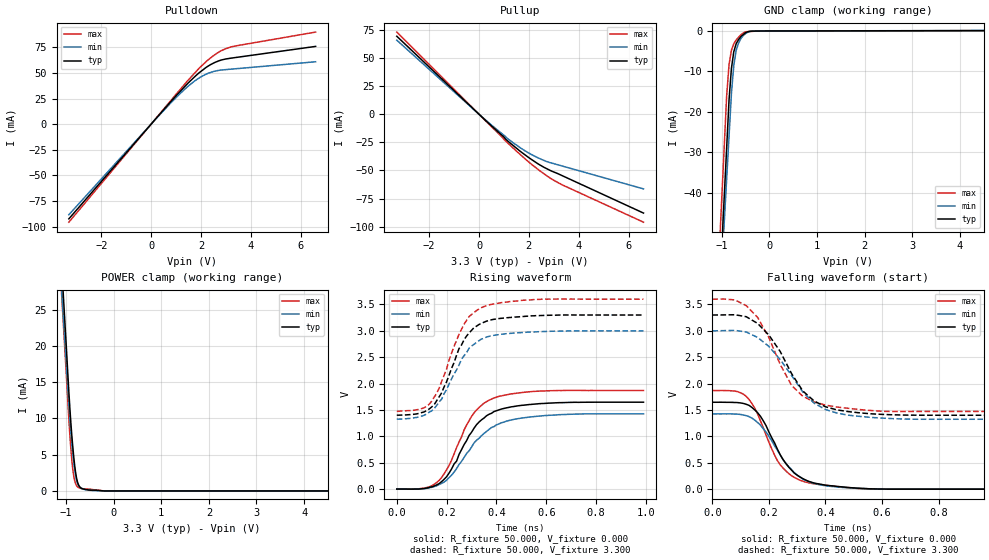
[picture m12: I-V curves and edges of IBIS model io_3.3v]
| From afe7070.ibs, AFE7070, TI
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[Model]   io_3.3v
Model_type I/O
Vinl=1.000E+00
Vinh=2.300E+00
Vref=0.000E+00
Rref=1.000E+06
Cref=0.000E+00
Vmeas=1.650E+00
C_comp   4.3600E-13   4.0000E-13   4.7200E-13
[Voltage Range]   3.300E+00   3.000E+00   3.600E+00
[POWER Clamp Reference]   3.300E+00   3.000E+00   3.600E+00
[GND Clamp Reference]   0.000E+00   0.000E+00   0.000E+00
[Pullup Reference]   3.300E+00   3.000E+00   3.600E+00
[Pulldown Reference]   0.000E+00   0.000E+00   0.000E+00
[Temperature Range]   25   85  -40
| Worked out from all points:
|   slope of the pulldown table from 0 to 0.495 V, typ, clamps not added: 35.8 ohm
|   slope of the pullup table from 0 to 0.495 V, typ, clamps not added: 48.5 ohm
|   GND clamp passes 1 mA (typ) near -0.56 V on its own axis
|   POWER clamp passes 1 mA (typ) near -0.75 V on its own axis
|   rising waveform, R_fixture 50.000, V_fixture 0.000: 20-80 % time 128ps typ, 149ps min, 118ps max; typ from 0 V to 1.65 V
|   falling waveform, R_fixture 50.000, V_fixture 0.000: 20-80 % time 108ps typ, 115ps min, 101ps max; typ from 1.65 V to 0 V
|   rising waveform, R_fixture 50.000, V_fixture 3.300: 20-80 % time 109ps typ, 118ps min, 108ps max; typ from 1.4 V to 3.3 V
|   falling waveform, R_fixture 50.000, V_fixture 3.300: 20-80 % time 137ps typ, 148ps min, 125ps max; typ from 3.3 V to 1.4 V
[GND Clamp]
-3.3V     -598.8mA   -544.4mA   -610mA
-900mV    -29mA      -36.72mA   -16.07mA
-850mV    -17.13mA   -26.15mA   -8.365mA
-800mV    -9.303mA   -15.57mA   -4.792mA
-750mV    -5.128mA   -8.543mA   -3.172mA
-700mV    -3.157mA   -4.777mA   -2.199mA
-650mV    -2.135mA   -2.997mA   -1.566mA
-600mV    -1.36mA    -1.854mA   -932uA
-500mV    -399uA     -615.8uA   -196.2uA
-400mV    -50.66uA   -108.8uA   -123.4uA
-175mV    -5.712uA   -4.952uA   -12.66uA
6.6V      127.9uA    166.2uA    116.8uA
[Power Clamp]
-3.3V     283.4mA    254.2mA    276.7mA
-1.02V    22.77mA    20.23mA    18.9mA
-920mV    11.43mA    10.06mA    7.72mA
-880mV    7.747mA    6.684mA    4.33mA
-860mV    6.2mA      5.228mA    3.077mA
-840mV    4.811mA    3.97mA     2.132mA
-800mV    2.561mA    2.114mA    1.016mA
-760mV    1.243mA    1.064mA    563.3uA
-720mV    622.7uA    586.8uA    407.3uA
-620mV    235.1uA    206.4uA    278uA
-200mV    0A         0A         0A
6.6V      0A         0A         0A
[Pullup]
-3.3V     69.46mA    65.96mA    73.14mA
340mV     -7.096mA   -6.576mA   -7.499mA
1.14V     -23.57mA   -21.53mA   -25.34mA
1.86V     -36.36mA   -32.74mA   -39.95mA
2.6V      -47.13mA   -41.02mA   -52.88mA
3.16V     -52.82mA   -44.96mA   -60.74mA
6.6V      -87.95mA   -66.43mA   -96.07mA
[Pulldown]
-3.3V     -92.37mA   -88.32mA   -95.62mA
800mV     22.26mA    21mA       23.29mA
1.44V     38.99mA    36.1mA     41.68mA
1.92V     50.01mA    44.98mA    54.35mA
2.24V     55.92mA    49.15mA    61.74mA
2.56V     60.25mA    51.72mA    67.83mA
2.84V     62.75mA    52.91mA    71.98mA
3.2V      64.39mA    53.67mA    75.33mA
6.6V      75.88mA    60.91mA    89.86mA
[Rising Waveform]
R_fixture = 50.000
V_fixture = 0.000
V_fixture_min = 0.000
V_fixture_max = 0.000
|  time   V(typ)   V(min)   V(max)
0s        46.74uV    11.3uV     188.6uV
110ps     9.836mV    8.726mV    19.34mV
170ps     103.4mV    86.13mV    163.8mV
210ps     303.8mV    216.8mV    449.4mV
300ps     1.076V     795.5mV    1.376V
330ps     1.27V      960.9mV    1.545V
390ps     1.469V     1.184V     1.726V
470ps     1.565V     1.321V     1.81V
590ps     1.623V     1.391V     1.859V
990ps     1.646V     1.425V     1.868V
[Falling Waveform]
R_fixture = 50.000
V_fixture = 0.000
V_fixture_min = 0.000
V_fixture_max = 0.000
|  time   V(typ)   V(min)   V(max)
0s        1.646V     1.425V     1.868V
90ps      1.64V      1.421V     1.846V
140ps     1.548V     1.347V     1.622V
180ps     1.296V     1.145V     1.164V
230ps     758.4mV    737.2mV    541.9mV
270ps     417.9mV    427.5mV    296.5mV
320ps     199.9mV    192.4mV    150.9mV
390ps     85.95mV    73.75mV    80.08mV
510ps     19.54mV    17mV       14.71mV
990ps     46.74uV    11.3uV     188.6uV
[Rising Waveform]
R_fixture = 50.000
V_fixture = 3.300
V_fixture_min = 3.000
V_fixture_max = 3.600
|  time   V(typ)   V(min)   V(max)
0s        1.4V       1.324V     1.473V
90ps      1.435V     1.372V     1.51V
140ps     1.555V     1.482V     1.665V
180ps     1.823V     1.703V     2.038V
230ps     2.399V     2.184V     2.708V
270ps     2.829V     2.528V     3.123V
290ps     2.958V     2.669V     3.267V
340ps     3.141V     2.843V     3.439V
560ps     3.287V     2.979V     3.595V
990ps     3.298V     2.998V     3.599V
[Falling Waveform]
R_fixture = 50.000
V_fixture = 3.300
V_fixture_min = 3.000
V_fixture_max = 3.600
|  time   V(typ)   V(min)   V(max)
0s        3.298V     2.998V     3.599V
80ps      3.304V     3.008V     3.585V
160ps     3.14V      2.874V     3.253V
200ps     2.918V     2.703V     2.871V
240ps     2.608V     2.454V     2.361V
280ps     2.19V      2.155V     1.967V
320ps     1.86V      1.84V      1.759V
400ps     1.561V     1.509V     1.593V
520ps     1.446V     1.379V     1.508V
3.96ns    1.4V       1.324V     1.473V
[Ramp]
dV/dt_r   9.6100E-01/1.2760E-10  8.5600E-01/1.4940E-10  1.1039E+00/1.2271E-10
dV/dt_f   1.1400E+00/1.3350E-10  1.0050E+00/1.4660E-10  1.2769E+00/1.2553E-10
R_load = 50
